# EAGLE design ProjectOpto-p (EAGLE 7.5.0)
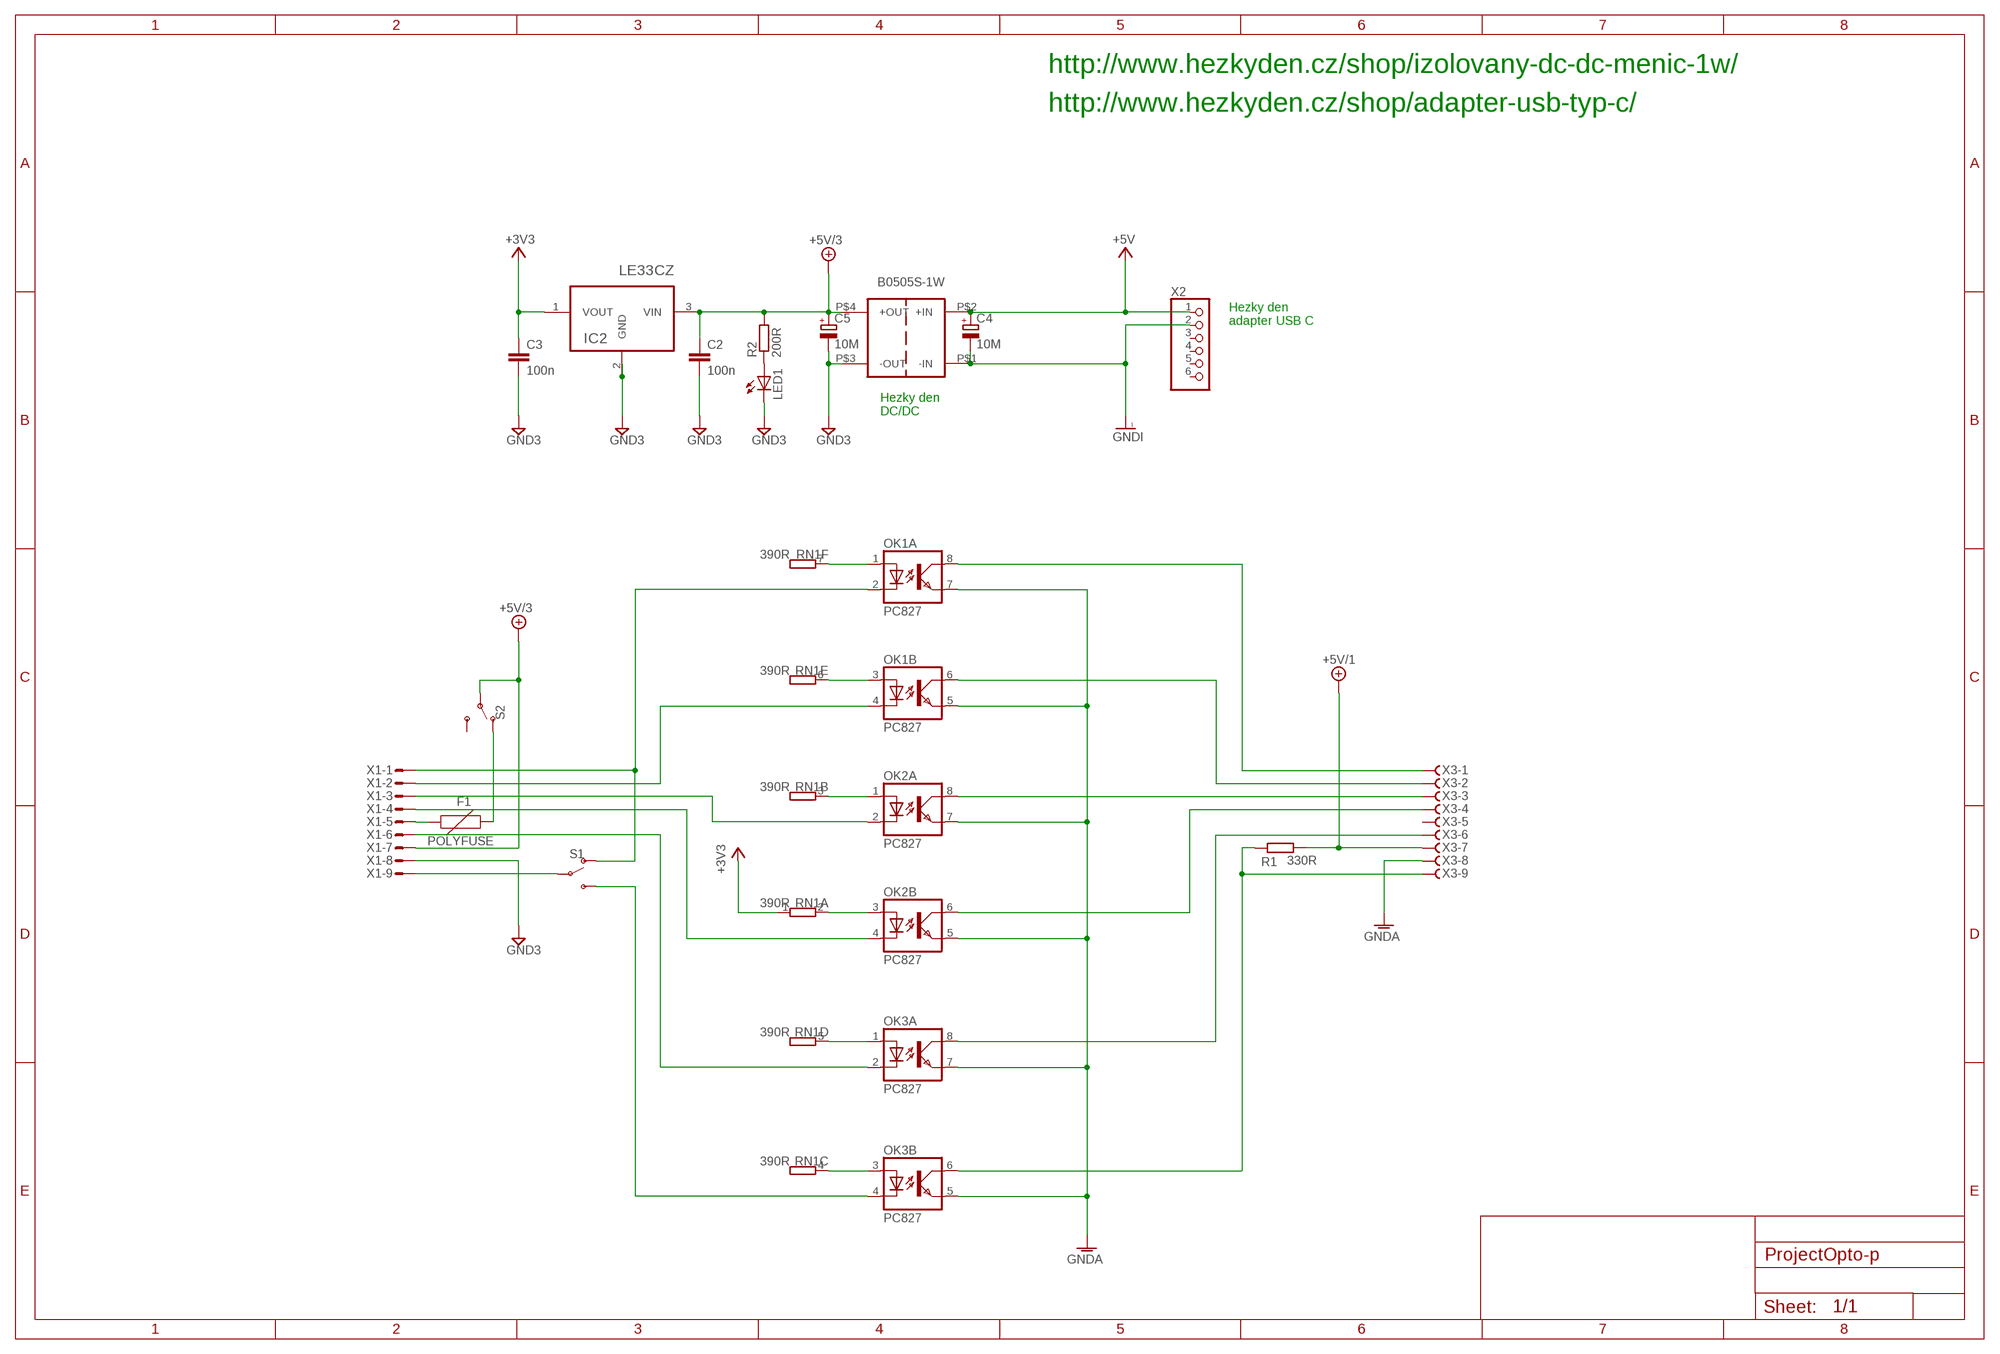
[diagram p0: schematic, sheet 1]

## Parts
B0505S-1W  BXXXXS  [BXXXXS]
C2  100n  C-EU025-024X044  [C025-024X044]
C3  100n  C-EU025-024X044  [C025-024X044]
C4  10M  CPOL-EUE2-4  [E2-4]
C5  10M  CPOL-EUE2-4  [E2-4]
F1  POLYFUSE  PPTC_PTH  [PTH]
IC2  LE33CZ  [TO127P254X749-3]
LED1  LED3MM  [LED3MM]
OK1  PC827  [DIL08]
OK2  PC827  [DIL08]
OK3  PC827  [DIL08]
R1  330R  R-EU_0204/7  [0204/7]
R2  200R  R-EU_0204/7  [0204/7]
RN1  390R  GE06R  [SIL7]
S1  SWITCH-SPDT-PTH-11.6X4.0MM  [SWITCH_SPDT_PTH_11.6X4.0MM]
S2  SWITCH-SPDT-PTH-11.6X4.0MM  [SWITCH_SPDT_PTH_11.6X4.0MM]
X1  M09DS  [M09D]
X2  PINHD-1X6  [1X06]
X3  F09DS  [F09D]

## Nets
+3V3: C3.1 IC2.1(VOUT) RN1.1
+5V: B0505S-1W.P$2(+IN) C4.+ X2.1
+5V/1: R1.2 X3.7
+5V/3: B0505S-1W.P$4(+OUT) C2.1 C5.+ IC2.3(VIN) R2.2 S2.2(P) X1.7
ADOWN: OK1.6(B:COL) X3.2
AFIRE: OK3.8(A:COL) X3.6
AFIREB: OK3.6(B:COL) R1.1 X3.9
ALEFT: OK2.8(A:COL) X3.3
ARIGHT: OK2.6(B:COL) X3.4
AUP: OK1.8(A:COL) X3.1
DOWN: OK1.4(B:C) X1.2
GND3: B0505S-1W.P$3(-OUT) C2.2 C3.2 C5.- IC2.2(GND) LED1.K(C) X1.8
GNDA: OK1.5(B:EMIT) OK1.7(A:EMIT) OK2.5(B:EMIT) OK2.7(A:EMIT) OK3.5(B:EMIT) OK3.7(A:EMIT) X3.8
GNDI: B0505S-1W.P$1(-IN) C4.- X2.2
LEFT: OK2.2(A:C) X1.3
N$2: LED1.A R2.1
N$3: S1.2(P) X1.9
N$4: OK3.1(A:A) RN1.5
N$5: OK3.3(B:A) RN1.4
N$6: OK2.1(A:A) RN1.3
N$7: OK2.3(B:A) RN1.2
N$8: OK1.1(A:A) RN1.7
N$9: OK1.3(B:A) RN1.6
N$10: F1.P$1 X1.5
N$12: F1.P$2 S2.1(O)
N$31: OK3.2(A:C) X1.6
N$32: OK3.4(B:C) S1.3(S)
RIGHT: OK2.4(B:C) X1.4
UP: OK1.2(A:C) S1.1(O) X1.1
Unconnected: S2.3(S) X2.3 X2.4 X2.5 X2.6 X3.5

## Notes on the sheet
- http://www.hezkyden.cz/shop/izolovany-dc-dc-menic-1w/
- http://www.hezkyden.cz/shop/adapter-usb-typ-c/
- Hezky den
  adapter USB C
- Hezky den
  DC/DC

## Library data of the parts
B0505S-1W = BXXXXS:BXXXXS
C2 C3 = rcl:C-EU: CAPACITOR, European symbol
C4 C5 = rcl:CPOL-EU: POLARIZED CAPACITOR, European symbol
F1 = SparkFun-Fuses:PPTC: Resettable Fuse PPTC; PROD_ID: RES-08490; VALUE: 72V/0.25A
IC2 = LE33CZ:LE33CZ: Check availability; AVAILABILITY: In Stock; CHECK_PRICES: https://www.snapeda.com/parts/LE33CZ/STMicroelectronics/view-part/?ref=eda; DESCRIPTION: Linear Voltage Regulator IC Positive Fixed 1 Output 100mA TO-92-3; MF: STMicroelectronics; MP: LE33CZ; PACKAGE: TO-92 STMicroelectronics; PRICE: None; SNAPEDA_LINK: https://www.snapeda.com/parts/LE33CZ/STMicroelectronics/view-part/?ref=snap
LED1 = led:LED: LED
OK1-OK3 = optocoupler:PC827: SHARP OPTO COUPLER; OC_FARNELL: unknown; OC_NEWARK: unknown
R1 R2 = rcl:R-EU_: RESISTOR, European symbol
RN1 = resistor-sil:GE06R: SIL RESISTOR; OC_FARNELL: unknown; OC_NEWARK: unknown
S1 S2 = SparkFun-Switches:SWITCH-SPDT: Single Pole, Double Throw (SPDT) Switch Single-pole, double-throw (SPDT) switch. Variant Overview SMD-AYZ0202 Surface Mount DPDT Switch (COM-00597) Used on e.g. LilyPad Arduino USB - ATmega32U4 Board PTH-11.6X4.0MM SPDT Mini Power Switch (COM-00102) Used on e.g. SparkFun Simon Says - Through-Hole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; PROD_ID: SWCH-08261; SF_SKU: COM-00102
X1 = con-subd:M09?S: SUB-D; OC_FARNELL: unknown; OC_NEWARK: unknown
X2 = pinhead:PINHD-1X6: PIN HEADER
X3 = con-subd:F09?S: SUB-D; OC_FARNELL: unknown; OC_NEWARK: unknown

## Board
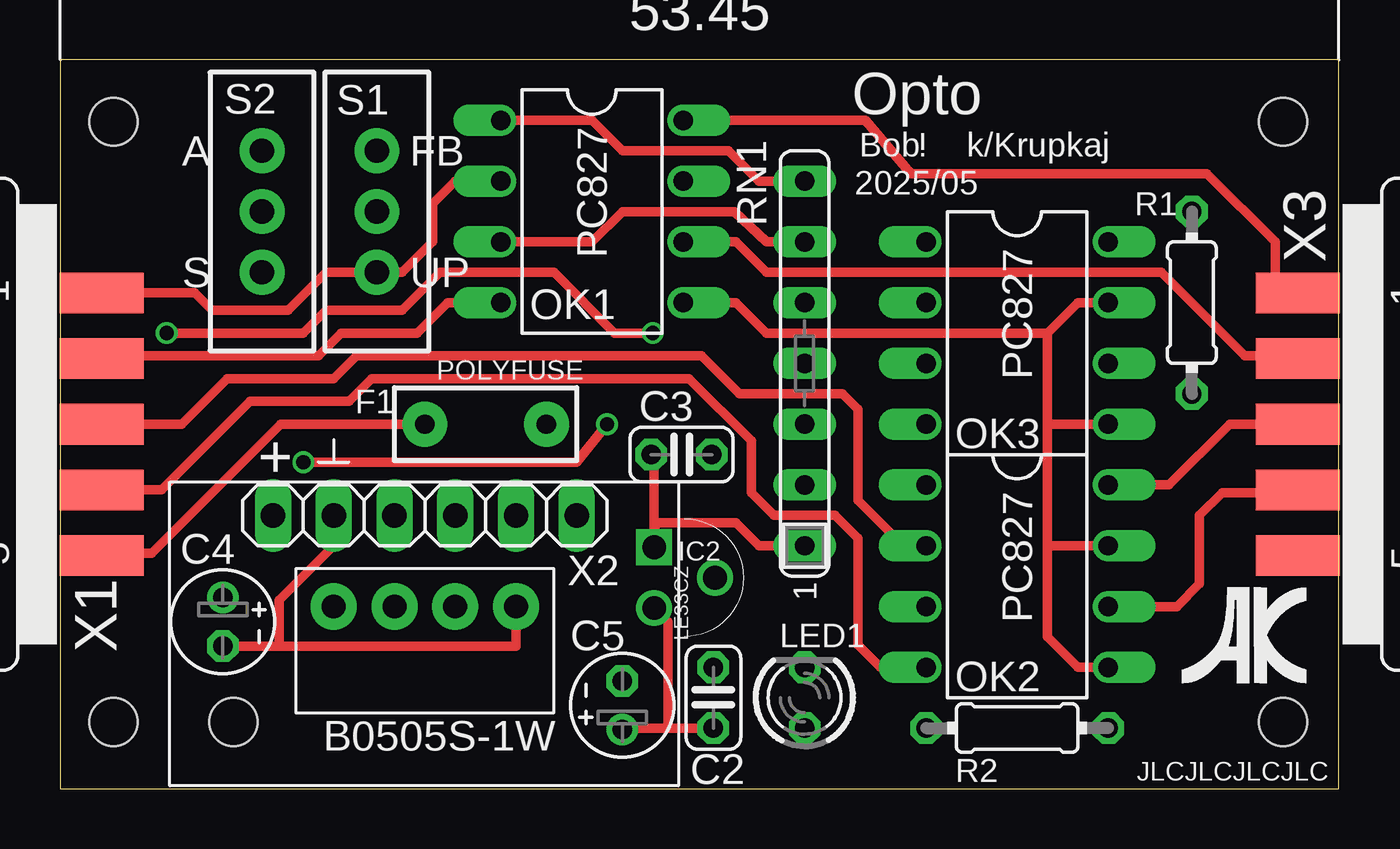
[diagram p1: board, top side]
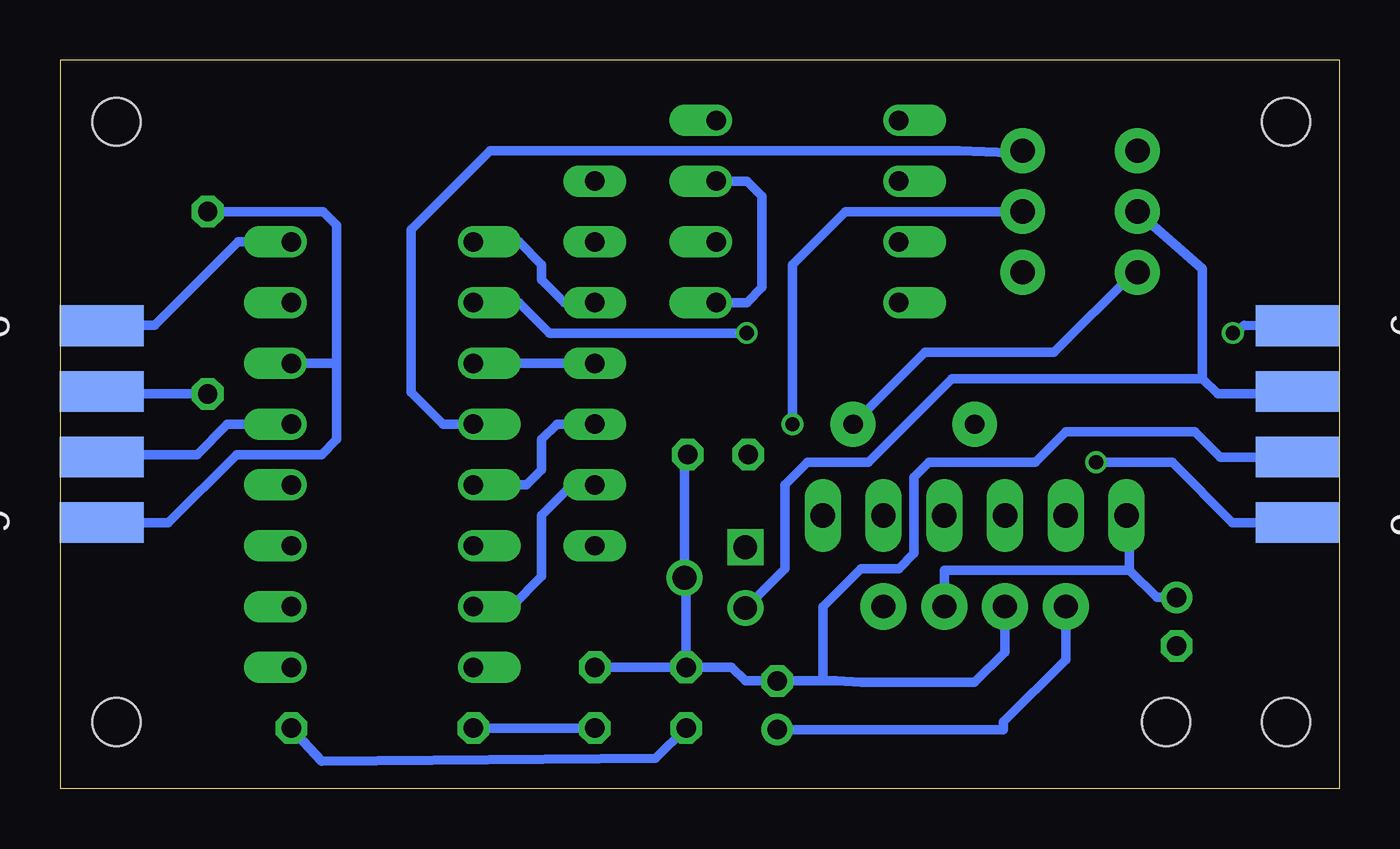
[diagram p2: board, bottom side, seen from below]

Size 53.45 x 30.47 mm. Coordinates in mm from the lower left corner, seen from the top.
Outline: 0,0 53.45,0 53.45,30.47 0,30.47 0,0
Copper layers (1*16): Top 0.035mm / dielectric 1.5mm / Bottom 0.035mm
Design rules "SeeedStudio_2layer_DRU_no_angle_20140221": minimum track width 6mil, minimum drill 12mil, track to track 6mil, track to pad 6mil, pad to pad 6mil, via to via 6mil, smd to smd 0mil, copper to edge 10mil, drill to drill 10mil, minimum pad ring 10mil, minimum via ring 6mil, stop-mask expansion 2mil, vias tented up to drill 100mil, thermal gap 10mil
Holes 2 mm at 51.12,27.88 51.12,2.79 7.24,2.79 2.22,27.88 2.22,2.79

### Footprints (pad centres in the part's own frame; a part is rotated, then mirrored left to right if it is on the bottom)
BXXXXS = drill 1 pad 1.93: P$1 -3.81,0; P$2 -1.27,0; P$3 1.27,0; P$4 3.81,0
C025-024X044 = drill 0.813 octagon: 1 -1.27,0; 2 1.27,0
E2-4 = drill 0.813 pad 1.27: + -1.016,0 | drill 0.813 pad 1.27 octagon: - 1.016,0
PTH = drill 0.8 pad 1.88: P$1 -2.54,0; P$2 2.54,0
TO127P254X749-3 = drill 0.991 square: 1 -2.54,-2.54 | drill 0.991: 2 -1.27,0; 3 0,-2.54
LED3MM = drill 0.813 octagon: A -1.27,0; K 1.27,0
DIL08 = drill 0.813 offset: 1 -3.81,-3.81; 2 -1.27,-3.81; 3 1.27,-3.81; 4 3.81,-3.81; 5 3.81,3.81; 6 1.27,3.81; 7 -1.27,3.81; 8 -3.81,3.81
0204/7 = drill 0.813 octagon: 1 -3.81,0; 2 3.81,0
SIL7 = drill 0.813 long: 1 -7.62,0; 2 -5.08,0; 3 -2.54,0; 4 0,0; 5 2.54,0; 6 5.08,0; 7 7.62,0
SWITCH_SPDT_PTH_11.6X4.0MM = drill 1.016 pad 1.88: 1 0,2.54; 2 0,0; 3 0,-2.54
M09D = smd 1.7 x 3.5: 1 5.486,-6.045; 2 2.743,-6.045; 3 0,-6.045; 4 -2.743,-6.045; 5 -5.486,-6.045 | smd 1.7 x 3.5 bottom: 6 4.115,-6.045; 7 1.372,-6.045; 8 -1.372,-6.045; 9 -4.115,-6.045
1X06 = drill 1.016 long: 1 -6.35,0; 2 -3.81,0; 3 -1.27,0; 4 1.27,0; 5 3.81,0; 6 6.35,0
F09D = smd 1.7 x 3.5: 1 -5.486,-6.045; 2 -2.743,-6.045; 3 0,-6.045; 4 2.743,-6.045; 5 5.486,-6.045 | smd 1.7 x 3.5 bottom: 6 -4.115,-6.045; 7 -1.372,-6.045; 8 1.372,-6.045; 9 4.115,-6.045

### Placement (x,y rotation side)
B0505S-1W  15.24,7.62 180 top
C2  27.31,3.81 90 top
C3  25.97,13.97 0 top
C4  6.79,6.98 270 top
C5  23.5,3.49 90 top
F1  17.78,15.24 0 top
IC2  27.37,7.56 270 top
LED1  31.11,3.81 90 top
OK1  22.22,24.13 270 top
OK2  40,8.89 270 top
OK3  40,19.05 270 top
R1  47.31,20.32 270 top
R2  40,2.54 0 top
RN1  31.11,17.78 90 top
S1  13.23,24.13 180 top
S2  8.43,24.13 180 top
X1  -4.32,15.24 90 top
X2  15.24,11.43 0 top
X3  57.79,15.24 270 top

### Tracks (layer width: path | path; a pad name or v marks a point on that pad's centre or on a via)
+3V3
  Top 0.406: RN1.1 29.21,10.16 28.26,11.11 24.89,11.11 IC2.1 24.83,13.53 C3.1
+5V
  Bottom 0.406: X2.1 8.76,11.3 8.76,9.14 | 8.76,9.14 7.62,8 C4.+ | 8.76,9.14 15.24,9.14 16.45,9.14 16.51,9.14 B0505S-1W.P$2
+5V/1
  Bottom 0.406: X3.7 51,16.51 R1.2
+5V/3
  Top 0.406: C2.1 25.4,2.54 | IC2.3 25.4,6.98 25.4,2.54 | 25.4,2.54 23.56,2.54 C5.+
  Bottom 0.406: C2.1 28.57,1.27 42.54,1.14 R2.2 | C5.+ 14.03,2.48 14.03,2.79 11.43,5.4 B0505S-1W.P$4 | S2.2 5.71,21.73 5.71,17.14 | 5.71,17.14 16.19,17.14 19.68,13.65 22.22,13.65 23.18,12.7 23.18,9.21 IC2.3 24.45,7.62 | 5.71,17.14 5.08,16.51 1.83,16.51 X1.7
ADOWN
  Top 0.406: X3.2 50.99,18.1 49.53,18.1 46.04,21.59 29.53,21.59 28.26,22.86 OK1.6
AFIRE
  Bottom 0.406: X3.6 51.09,19.37 49.53,19.37 46.04,22.86 OK3.8
AFIREB
  Bottom 0.406: X3.9 51.09,11.11 48.96,11.11 46.1,13.97 42.54,13.97 41.91,14.6 41.91,17.78 | 41.91,17.78 OK3.6 | 41.91,17.78 41.91,23.56 42.48,24.13 R1.1
ALEFT
  Top 0.406: OK2.8 46.35,12.7 48.9,15.24 X3.3
ARIGHT
  Top 0.406: X3.4 50.99,12.38 48.58,12.38 47.63,11.43 47.63,8.57 46.67,7.62 OK2.6
AUP
  Top 0.406: X3.1 50.8,21.03 50.8,22.86 47.94,25.72 35.56,25.72 33.65,27.94 OK1.8
DOWN
  Top 0.406: X1.2 2.35,18.1 10.8,18.1 11.75,19.05 14.92,19.05 16.19,20.32 OK1.4
GND3
  Bottom 0.406: LED1.K C2.2 | 21.59,4.51 21.02,4.51 20,4.45 15.24,4.45 13.97,5.71 B0505S-1W.P$3 | 21.59,4.51 C5.- 24.83,4.51 25.4,5.08 C2.2 | C2.2 27.31,8.57 IC2.2 27.37,13.84 C3.2 | X1.8 4.98,13.87 6.03,14.92 11.43,14.92 12.7,13.65 17.14,13.65 17.78,13.02 17.78,9.84 18.42,9.21 20,9.21 21.59,7.62 21.59,4.51
GNDA
  Top 0.406: OK2.5 42.54,5.08 41.28,6.35 41.28,10.16 | 41.28,10.16 OK2.7 | 41.28,19.05 41.28,15.24 | 41.28,15.24 41.28,10.16 | OK3.5 41.28,15.24 | OK1.5 28.26,20.32 29.53,19.05 41.28,19.05 | 41.28,19.05 42.54,20.32 OK3.7
  Bottom 0.406: X3.8 51,13.97 47.75,13.97 46.48,15.24 OK3.5 | OK1.7 24.77,25.4 24.13,24.77 24.13,20.95 24.77,20.32 OK1.5
GNDI
  Top 0.406: X2.2 11.43,10.16 9.14,7.87 9.14,6.03 9.21,5.97 | C4.- 9.21,5.97 | 9.21,5.97 19.05,5.97 B0505S-1W.P$1
LEFT
  Top 0.406: OK2.2 35.24,10.16 33.34,12.06 33.34,15.88 32.7,16.51 28.38,16.51 26.8,18.1 12.38,18.1 11.43,17.14 6.98,17.14 5.08,15.24 X1.3
N$2
  Bottom 0.406: R2.1 LED1.A
N$3  (via drill 0.6)
  Top 0.406: v10.16,13.65 21.59,13.65 v22.86,15.24
  Bottom 0.406: X1.9 4.46,11.12 6.98,13.65 v10.16,13.65 | v22.86,15.24 22.86,21.91 20.64,24.13 S1.2
N$4
  Bottom 0.406: RN1.5 32.39,20.32 33.34,21.27 33.34,21.91 34.29,22.86 OK3.1
N$5
  Bottom 0.406: RN1.4 OK3.3
N$6
  Bottom 0.406: RN1.3 32.7,15.24 33.34,14.6 33.34,13.34 33.97,12.7 OK2.1
N$7
  Bottom 0.406: RN1.2 32.07,12.7 33.34,11.43 33.34,8.89 34.61,7.62 OK2.3
N$8
  Top 0.406: OK1.1 22.22,27.94 23.5,26.67 27.94,26.67 29.21,25.4 RN1.7
N$9
  Top 0.406: RN1.6 29.53,22.86 28.19,24.13 23.5,24.13 22.22,22.86 OK1.3
N$10
  Top 0.406: X1.5 1.82,9.84 3.81,9.84 9.21,15.24 F1.P$1
N$12
  Bottom 0.406: F1.P$2 17.32,18.24 11.93,18.24 8.57,21.59 S2.1
N$31  (via drill 0.6)
  Top 0.406: v24.77,19.05 23.18,19.05 20.64,21.59 15.88,21.59 14.29,20 11.11,20 10.16,19.05 v4.44,19.05
  Bottom 0.406: OK3.2 34.29,20.32 33.02,19.05 v24.77,19.05 | v4.44,19.05 3.96,19.37 X1.6
N$32
  Bottom 0.406: OK3.4 37.46,15.24 38.8,16.57 38.8,23.37 35.5,26.67 15.88,26.67 13.23,26.57 S1.3
RIGHT
  Top 0.406: OK2.4 34.29,5.08 33.34,6.03 33.34,10.48 32.39,11.43 29.85,11.43 28.89,12.38 28.89,14.54 26.29,17.14 13.02,17.14 12.07,16.19 7.94,16.19 4.24,12.5 X1.4 1.93,12.7
UP
  Top 0.406: OK1.2 16.51,25.4 15.56,24.45 15.56,22.86 14.29,21.59 S1.1 11.11,21.59 9.53,20 6.35,20 5.63,20.73 X1.1

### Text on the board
tPlace: Opto | Bob | ! | k/Krupkaj | 2025/05
tNames: A | FB | S | UP | + | JLCJLCJLCJLC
